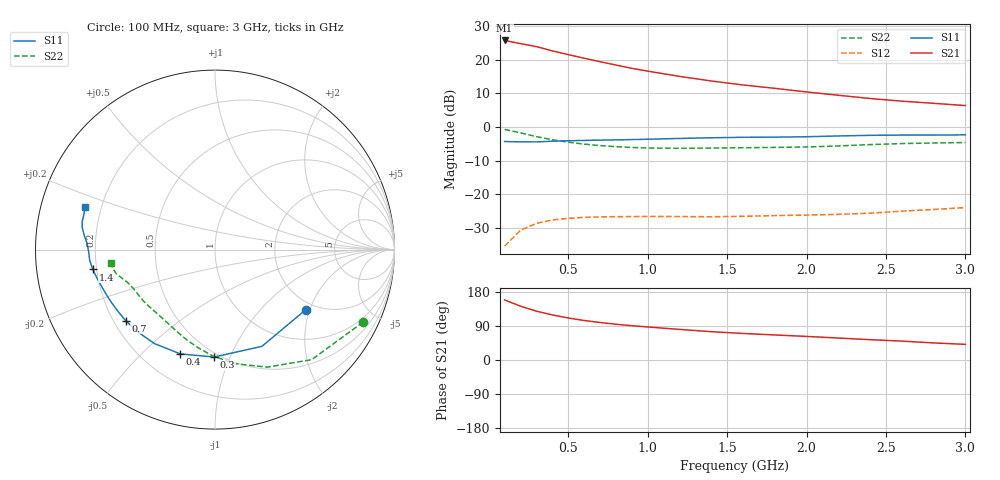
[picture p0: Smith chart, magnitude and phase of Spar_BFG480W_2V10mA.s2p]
! Filename: 210BFG480.001
! Title: BFG480W
! Bias: Vce=2V; Ic=10mA
! Company: NXP Semiconductors NL
! User: Quality&Reliability T&D
! Measure time: 10 Nov 1999 / 11:53:15
#  MHz  S  MA  R 50
! Freq  S11  S21  S12  S22  :
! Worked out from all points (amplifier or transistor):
!   20 points, 100 MHz to 3 GHz, reference 50 ohm
!   highest |S21| = 25.7 dB at 100 MHz (marker M1)
!   |S21| within 3 dB of that: start of sweep to 392.1 MHz
!   unconditionally stable (mu >= 1): 1.741 GHz to end of sweep
!   at 400 MHz: K = 0.22, MSG = 25.2 dB, |S12| = -27.7 dB
!   at 1.2 GHz: K = 0.71, MSG = 20.9 dB, |S12| = -26.7 dB
!   at 3 GHz: K = 1.24, MAG = 12.2 dB, |S12| = -24.0 dB
!   S11 on the Smith chart (normalised r, x): 100 MHz: 1.77, -1.88; 300 MHz: 0.47, -0.87; 400 MHz: 0.35, -0.66; 700 MHz: 0.25, -0.33; 1.4 GHz: 0.18, -0.08; 3 GHz: 0.14, +0.15
100  0.6064 -33.5  19.35 158.4  0.01681 70.9  0.9188 -26.1
200  0.5991 -64.1  17.36 142.0  0.02905 56.1  0.8163 -48.7
300  0.5984 -90.5  15.68 128.9  0.03671 46.0  0.7167 -66.0
400  0.6123 -108.4  13.54 119.0  0.04125 38.8  0.6466 -79.7
500  0.6229 -122.8  11.92 110.9  0.04363 34.0  0.5935 -91.0
600  0.6296 -133.6  10.54 104.2  0.04506 30.8  0.5548 -99.8
700  0.6362 -141.6  9.342 99.0  0.04583 28.9  0.5277 -107.1
800  0.6414 -148.1  8.347 94.4  0.04623 27.7  0.508 -113.2
900  0.648 -153.1  7.453 90.6  0.04631 27.2  0.4947 -118.6
1000  0.6558 -157.8  6.769 87.2  0.04652 27.2  0.4858 -123.6
1200  0.6734 -165.3  5.655 80.8  0.04637 27.9  0.4804 -132.1
1400  0.6898 -170.8  4.831 74.7  0.0461 29.7  0.4846 -138.9
1600  0.7007 -175.1  4.214 70.0  0.04668 32.9  0.4906 -144.1
1800  0.7044 -179.2  3.752 66.1  0.04795 36.7  0.4956 -149.2
2000  0.7143 177.1  3.316 62.2  0.04881 40.8  0.5031 -154.5
2200  0.734 173.6  2.958 57.9  0.04997 44.2  0.521 -159.5
2400  0.7497 170.6  2.65 53.6  0.0521 47.4  0.5454 -163.4
2600  0.7565 168.0  2.418 49.9  0.05582 50.5  0.5657 -166.1
2800  0.756 165.2  2.246 45.1  0.05909 52.2  0.5765 -169.0
3000  0.7619 162.1  2.079 41.3  0.06301 54.3  0.5858 -172.5
